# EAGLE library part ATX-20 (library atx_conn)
ATX PC-Motherboard Power connector
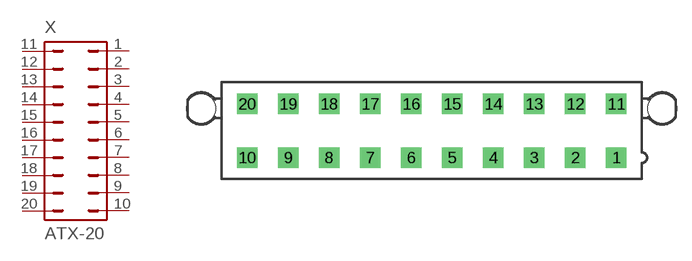
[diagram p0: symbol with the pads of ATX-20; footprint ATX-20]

Designator prefix X

## ATX-20  [ATX-20]
1  1  pas
2  2  pas
3  3  pas
4  4  pas
5  5  pas
6  6  pas
7  7  pas
8  8  pas
9  9  pas
10  10  pas
11  11  pas
12  12  pas
13  13  pas
14  14  pas
15  15  pas
16  16  pas
17  17  pas
18  18  pas
19  19  pas
20  20  pas

## Footprint ATX-20 (pad centres in mm)
Mini FIT connector 20 pol ATX PC-Motherboard Power connector Source: http://www.molex.com
drill 1.4 square: 1 18.9,-2.75; 2 14.7,-2.75; 3 10.5,-2.75; 4 6.3,-2.75; 5 2.1,-2.75; 6 -2.1,-2.75; 7 -6.3,-2.75; 8 -10.5,-2.75; 9 -14.7,-2.75; 10 -18.9,-2.75; 11 18.9,2.75; 12 14.7,2.75; 13 10.5,2.75; 14 6.3,2.75; 15 2.1,2.75; 16 -2.1,2.75; 17 -6.3,2.75; 18 -10.5,2.75; 19 -14.7,2.75; 20 -18.9,2.75
hole 3 at 23.6,2.29
hole 3 at -23.6,2.29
